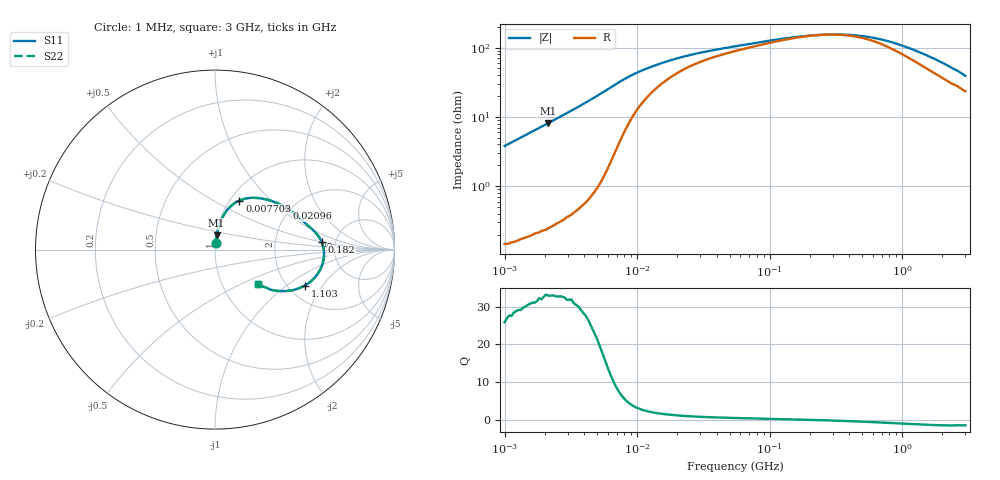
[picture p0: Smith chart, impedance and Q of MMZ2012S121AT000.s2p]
! S-parameter Generated by TDK Corporation
! Copyright(C) 2016 TDK Corporation.
! All Rights Reserved.
! TDK P/N: MMZ2012S121AT000 (Chip Beads)
! Property: |Z|=120¶ at 100MHz
! Size(LxWxT): 2x1.25x0.85mm, 0.079x0.049x0.033inches
! Model Type: s2p (Touchstone File Format Version 1.0)
! Frequency: DC=Yes Start=1MHz Stop=3000MHz 202points Log-sweep
! Note: This model was converted from impedance.
! Model Generated on May. 16, 2016
! Hash(MD5):
! Port Assignments:
!  1 ---@@@--- 2
! Applicable Conditions:
!  Temperature = 25 degC
!  DC Bias Current = 0 A
!  Small Signal Operation
! Terms and conditions regarding TDK Simulation Models
! (1)This simulation model is being provided solely for informational purposes. Please refer to the specifications of the products in terms of detailed characteristics of such products.
! (2)In no event shall TDK Corporation of any of its subsidiaries be liable for any loss or damage arising, directly or indirectly,
!  From any information contained in this simulation model, including, but not limited to loss or damages arising from any inaccuracies, omissions or errors in connection with such information.
! (3)Any and all copyrights on this simulation model are owned by TDK Corporation.
!  Duplication or redistribution of this simulation model without prior written permission from TDK Corporation is prohibited.
! (4)This simulation model is subject to any modification or change without any prior notice.
! (5)Neither TDK Corporation nor any of its subsidiaries shall make any warranty, express or implied,
!  Including but not limited to the correctness, implied warranties of merchantability and fitness for a particular purpose with respect to this simulation models.
! (6)The use of this simulation model shall be deemed to have consented to the terms and conditions hereof.
# MHz S MA R 50
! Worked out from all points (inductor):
!   201 points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, 1 MHz to 3 GHz, reference 50 ohm
!   read as one part in series: L = 604 nH near 1.041 MHz
!   highest Q = 32.9 at 2.14 MHz (marker M1), where L = 606 nH
!   self-resonance near 262.8 MHz
!   S11 on the Smith chart (normalised r, x): 1 MHz: 1.00, +0.08; 7.703 MHz: 1.10, +0.66; 20.96 MHz: 1.90, +1.11; 182 MHz: 3.89, +0.49; 1.103 GHz: 2.45, -1.38; 3 GHz: 1.47, -0.63
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1  0.03792 85.6  0.9978 -2.2  0.9978 -2.2  0.03792 85.6
2.13957  0.08105 83.6  0.9942 -4.6  0.9942 -4.6  0.08105 83.6
3.900413  0.1499 79.4  0.9834 -8.6  0.9834 -8.6  0.1499 79.4
5.592179  0.2213 73.8  0.9621 -12.8  0.9621 -12.8  0.2213 73.8
7.703107  0.3049 63.6  0.9063 -17.5  0.9063 -17.5  0.3049 63.6
10.19448  0.3661 52.0  0.8263 -20.4  0.8263 -20.4  0.3661 52.0
14.61624  0.4208 39.5  0.7264 -21.6  0.7264 -21.6  0.4208 39.5
20.95589  0.4612 30.0  0.6436 -21.0  0.6436 -21.0  0.4612 30.0
31.27247  0.4935 22.4  0.5755 -19.1  0.5755 -19.1  0.4935 22.4
54.77226  0.5303 15.4  0.5085 -16.1  0.5085 -16.1  0.5303 15.4
108.1723  0.5723 8.9  0.4436 -11.5  0.4436 -11.5  0.5723 8.9
182.0241  0.5963 3.9  0.407 -5.7  0.407 -5.7  0.5963 3.9
213.6344  0.6012 2.2  0.3999 -3.3  0.3999 -3.3  0.6012 2.2
318.8066  0.6081 -2.2  0.3931 3.4  0.3931 3.4  0.6081 -2.2
439.1493  0.6064 -6.2  0.4025 9.4  0.4025 9.4  0.6064 -6.2
581.181  0.5981 -10.3  0.4253 14.6  0.4253 14.6  0.5981 -10.3
800.5644  0.5767 -15.7  0.4716 19.4  0.4716 19.4  0.5767 -15.7
1102.76  0.5387 -21.8  0.5386 21.8  0.5386 21.8  0.5387 -21.8
1459.42  0.49 -27.4  0.6081 21.7  0.6081 21.7  0.49 -27.4
1931.433  0.4279 -32.7  0.6801 19.8  0.6801 19.8  0.4279 -32.7
2660.507  0.3431 -37.3  0.7561 16.0  0.7561 16.0  0.3431 -37.3
3000  0.3072 -38.9  0.7851 14.2  0.7851 14.2  0.3072 -38.9
